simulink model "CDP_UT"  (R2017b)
settings: Solver=FixedStepDiscrete  StartTime=0.0  StopTime=10.0  FixedStep=0.01  RelTol=1e-3  EnableMultiTasking=on
undefined symbols (not defined in the file): ASWTYPE_FALSE, ASWTYPE_TRUE, CaCDP_CellTempNTCVoltTable_mV, CaCDP_CellTempTable_C, CaCDP_CMUPCBTempNTCVoltTable_mV, CaCDP_CMUPCBTempTable_C, CbCDP_DiffBusbarTempStateCheck_flg, CbCDP_DiffCellTempStateCheck_flg, CbCDP_DiffCellVoltStateCheck_flg, CbCDP_IgnorUpdateVld_flg, CbCDP_MaxBusbarTempStateCheck_flg, CbCDP_MaxCellTempStateCheck_flg, CbCDP_MaxCellVoltStateCheck_flg, CbCDP_MinBusbarTempStateCheck_flg, CbCDP_MinCellTempStateCheck_flg, CbCDP_MinCellVoltStateCheck_flg, CcCDP_AFETempConfig_numb, CcCDP_AFETempFltThd_C, CcCDP_AFETempFltThdHys_C, CcCDP_BusbarTempRngFltHiThrd_C, CcCDP_BusbarTempRngFltLowThrd_C, CcCDP_CellDiffFltLevel1_mV, CcCDP_CellDiffFltLevel2_mV, CcCDP_CellDiffFltLevel3_mV, CcCDP_CellTempLowerLimit_C, CcCDP_CellTempRngFltHiThrd_C, CcCDP_CellTempRngFltLowThrd_C, CcCDP_CellTempUpperLimit_C, CcCDP_CellVoltConfig_numb, CcCDP_CellVoltLowerLimit_mV, CcCDP_CellVoltRngHiThrd_mV, CcCDP_CellVoltRngLowThrd_mV, CcCDP_CellVoltUpdateThrd_numb, CcCDP_CellVoltUpperLimit_mV, CcCDP_ChrgMaxCellTempFltLv1Thrd_C, CcCDP_ChrgMaxCellTempFltLv2Thrd_C, CcCDP_ChrgMaxCellTempFltLv3Thrd_C, CcCDP_ChrgMaxCellTempReturnDiff_C, CcCDP_ChrgMinCellTempFltLv1Thrd_C, CcCDP_ChrgMinCellTempFltLv2Thrd_C, CcCDP_ChrgMinCellTempFltLv3Thrd_C, CcCDP_ChrgMinCellTempReturnDiff_C, CcCDP_CMUPCBTempConfig_numb, CcCDP_CMUPCBTempFltThd_C, CcCDP_CMUPCBTempFltThdHys_C, CcCDP_DiffBusbarTempFltLevel1Thrd_C, CcCDP_DiffBusbarTempFltLevel2Thrd_C, CcCDP_DiffBusbarTempReturnDifference_C, CcCDP_DiffCellTempFltLevel1Thrd_C, CcCDP_DiffCellTempFltLevel2Thrd_C, CcCDP_DiffCellTempReturnDifference_C, CcCDP_DiffCellVoltReturnDifference_mV, CcCDP_DiffVoltCheckMaxCellTempCondition_C, CcCDP_DiffVoltCheckMaxCellVoltCondition_mV, CcCDP_DiffVoltCheckMinCellTempCondition_C, CcCDP_DiffVoltCheckMinCellVoltCondition_mV, CcCDP_DiffVoltCheckPackCurrCondition_A, CcCDP_MaxAFETempIniVal_C, CcCDP_MaxBusbarTempFltLevel1Thrd_C, CcCDP_MaxBusbarTempFltLevel2Thrd_C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
libraries: AIWAYS_Powertrain_BMS_lib x148, simulink x8
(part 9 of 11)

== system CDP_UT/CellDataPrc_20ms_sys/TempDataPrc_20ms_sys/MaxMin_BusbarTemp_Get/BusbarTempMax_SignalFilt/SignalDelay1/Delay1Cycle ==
  u : Inport
  Constant2 : Constant  Value=ASWTYPE_FALSE
  Switch : Switch  Criteria=u2 ~= 0  Threshold=1  RndMeth=Zero
  Unit Delay1 : UnitDelay  SampleTime=-1  StateName=StateName
  Unit Delay21 : UnitDelay  InitialCondition=1  SampleTime=-1  StateName=StateName
  y : Outport
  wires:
  Switch/1 -> y/1
  u/1 -> Switch/1, Unit Delay1/1
  Unit Delay1/1 -> Switch/3
  Unit Delay21/1 -> Switch/2
  Constant2/1 -> Unit Delay21/1

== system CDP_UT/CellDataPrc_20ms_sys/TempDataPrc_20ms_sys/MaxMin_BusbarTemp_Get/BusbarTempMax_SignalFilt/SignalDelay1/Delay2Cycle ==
  u : Inport
  Constant2 : Constant  Value=ASWTYPE_FALSE
  Switch : Switch  Criteria=u2 ~= 0  Threshold=1  RndMeth=Zero
  Unit Delay1 : UnitDelay  SampleTime=-1  StateName=StateName
  Unit Delay2 : UnitDelay  InitialCondition=1  SampleTime=-1  StateName=StateName
  Unit Delay21 : UnitDelay  InitialCondition=1  SampleTime=-1  StateName=StateName
  Unit Delay3 : UnitDelay  SampleTime=-1  StateName=StateName
  y : Outport
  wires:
  Unit Delay3/1 -> Switch/3
  Unit Delay2/1 -> Switch/2
  Constant2/1 -> Unit Delay21/1
  Unit Delay21/1 -> Unit Delay2/1
  Unit Delay1/1 -> Unit Delay3/1
  u/1 -> Unit Delay1/1, Switch/1
  Switch/1 -> y/1

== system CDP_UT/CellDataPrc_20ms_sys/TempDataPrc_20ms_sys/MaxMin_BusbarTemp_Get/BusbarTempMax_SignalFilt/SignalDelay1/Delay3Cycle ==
  u : Inport
  Constant2 : Constant  Value=ASWTYPE_FALSE
  Switch : Switch  Criteria=u2 ~= 0  Threshold=1  RndMeth=Zero
  Unit Delay1 : UnitDelay  SampleTime=-1  StateName=StateName
  Unit Delay2 : UnitDelay  InitialCondition=1  SampleTime=-1  StateName=StateName
  Unit Delay21 : UnitDelay  InitialCondition=1  SampleTime=-1  StateName=StateName
  Unit Delay3 : UnitDelay  SampleTime=-1  StateName=StateName
  Unit Delay4 : UnitDelay  InitialCondition=1  SampleTime=-1  StateName=StateName
  Unit Delay5 : UnitDelay  SampleTime=-1  StateName=StateName
  y : Outport
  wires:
  Unit Delay5/1 -> Switch/3
  Unit Delay4/1 -> Switch/2
  Unit Delay3/1 -> Unit Delay5/1
  Unit Delay2/1 -> Unit Delay4/1
  Constant2/1 -> Unit Delay21/1
  Unit Delay21/1 -> Unit Delay2/1
  Unit Delay1/1 -> Unit Delay3/1
  u/1 -> Unit Delay1/1, Switch/1
  Switch/1 -> y/1

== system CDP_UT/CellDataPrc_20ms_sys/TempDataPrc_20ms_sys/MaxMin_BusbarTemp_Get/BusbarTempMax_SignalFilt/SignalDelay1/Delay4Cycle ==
  u : Inport
  Constant2 : Constant  Value=ASWTYPE_FALSE
  Switch : Switch  Criteria=u2 ~= 0  Threshold=1  RndMeth=Zero
  Unit Delay{1,3,5,7} (4 alike) : UnitDelay  SampleTime=-1  StateName=StateName
  Unit Delay{2,4,6,21} (4 alike) : UnitDelay  InitialCondition=1  SampleTime=-1  StateName=StateName
  y : Outport
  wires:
  Unit Delay7/1 -> Switch/3
  Unit Delay6/1 -> Switch/2
  Unit Delay5/1 -> Unit Delay7/1
  Unit Delay4/1 -> Unit Delay6/1
  Unit Delay3/1 -> Unit Delay5/1
  Unit Delay2/1 -> Unit Delay4/1
  Constant2/1 -> Unit Delay21/1
  Unit Delay21/1 -> Unit Delay2/1
  Unit Delay1/1 -> Unit Delay3/1
  u/1 -> Unit Delay1/1, Switch/1
  Switch/1 -> y/1

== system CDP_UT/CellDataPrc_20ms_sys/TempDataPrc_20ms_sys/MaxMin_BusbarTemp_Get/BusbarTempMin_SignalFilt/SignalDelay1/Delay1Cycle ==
  u : Inport
  Constant2 : Constant  Value=ASWTYPE_FALSE
  Switch : Switch  Criteria=u2 ~= 0  Threshold=1  RndMeth=Zero
  Unit Delay1 : UnitDelay  SampleTime=-1  StateName=StateName
  Unit Delay21 : UnitDelay  InitialCondition=1  SampleTime=-1  StateName=StateName
  y : Outport
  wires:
  Constant2/1 -> Unit Delay21/1
  Unit Delay21/1 -> Switch/2
  Unit Delay1/1 -> Switch/3
  u/1 -> Unit Delay1/1, Switch/1
  Switch/1 -> y/1

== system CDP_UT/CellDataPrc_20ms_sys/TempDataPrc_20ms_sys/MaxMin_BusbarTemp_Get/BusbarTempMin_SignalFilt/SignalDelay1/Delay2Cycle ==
  u : Inport
  Constant2 : Constant  Value=ASWTYPE_FALSE
  Switch : Switch  Criteria=u2 ~= 0  Threshold=1  RndMeth=Zero
  Unit Delay1 : UnitDelay  SampleTime=-1  StateName=StateName
  Unit Delay2 : UnitDelay  InitialCondition=1  SampleTime=-1  StateName=StateName
  Unit Delay21 : UnitDelay  InitialCondition=1  SampleTime=-1  StateName=StateName
  Unit Delay3 : UnitDelay  SampleTime=-1  StateName=StateName
  y : Outport
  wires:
  Switch/1 -> y/1
  u/1 -> Switch/1, Unit Delay1/1
  Unit Delay1/1 -> Unit Delay3/1
  Unit Delay21/1 -> Unit Delay2/1
  Constant2/1 -> Unit Delay21/1
  Unit Delay2/1 -> Switch/2
  Unit Delay3/1 -> Switch/3

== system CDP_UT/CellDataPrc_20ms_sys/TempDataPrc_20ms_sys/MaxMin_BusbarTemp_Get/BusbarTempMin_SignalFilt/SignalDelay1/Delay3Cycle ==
  u : Inport
  Constant2 : Constant  Value=ASWTYPE_FALSE
  Switch : Switch  Criteria=u2 ~= 0  Threshold=1  RndMeth=Zero
  Unit Delay1 : UnitDelay  SampleTime=-1  StateName=StateName
  Unit Delay2 : UnitDelay  InitialCondition=1  SampleTime=-1  StateName=StateName
  Unit Delay21 : UnitDelay  InitialCondition=1  SampleTime=-1  StateName=StateName
  Unit Delay3 : UnitDelay  SampleTime=-1  StateName=StateName
  Unit Delay4 : UnitDelay  InitialCondition=1  SampleTime=-1  StateName=StateName
  Unit Delay5 : UnitDelay  SampleTime=-1  StateName=StateName
  y : Outport
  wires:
  Switch/1 -> y/1
  u/1 -> Switch/1, Unit Delay1/1
  Unit Delay1/1 -> Unit Delay3/1
  Unit Delay21/1 -> Unit Delay2/1
  Constant2/1 -> Unit Delay21/1
  Unit Delay2/1 -> Unit Delay4/1
  Unit Delay3/1 -> Unit Delay5/1
  Unit Delay4/1 -> Switch/2
  Unit Delay5/1 -> Switch/3

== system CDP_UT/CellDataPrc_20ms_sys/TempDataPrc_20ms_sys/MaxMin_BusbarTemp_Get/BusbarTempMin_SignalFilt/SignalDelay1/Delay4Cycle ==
  u : Inport
  Constant2 : Constant  Value=ASWTYPE_FALSE
  Switch : Switch  Criteria=u2 ~= 0  Threshold=1  RndMeth=Zero
  Unit Delay{1,3,5,7} (4 alike) : UnitDelay  SampleTime=-1  StateName=StateName
  Unit Delay{2,4,6,21} (4 alike) : UnitDelay  InitialCondition=1  SampleTime=-1  StateName=StateName
  y : Outport
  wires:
  Switch/1 -> y/1
  u/1 -> Switch/1, Unit Delay1/1
  Unit Delay1/1 -> Unit Delay3/1
  Unit Delay21/1 -> Unit Delay2/1
  Constant2/1 -> Unit Delay21/1
  Unit Delay2/1 -> Unit Delay4/1
  Unit Delay3/1 -> Unit Delay5/1
  Unit Delay4/1 -> Unit Delay6/1
  Unit Delay5/1 -> Unit Delay7/1
  Unit Delay6/1 -> Switch/2
  Unit Delay7/1 -> Switch/3

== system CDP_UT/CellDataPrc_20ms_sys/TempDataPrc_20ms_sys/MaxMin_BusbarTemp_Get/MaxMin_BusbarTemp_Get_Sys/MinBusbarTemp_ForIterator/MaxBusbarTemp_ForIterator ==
  LcCDP_IniOutputBusbarTemp_C : Inport
  LcCDP_IniOutputBusbarTempNumb_numb : Inport  Port=2
  LbCDP_IniOutputBusbarTempVld_flg : Inport  Port=3
  Constant3 : Constant  Value=CcCDP_MaxBusbarTempIniVal_C
  Logical Operator : Logic  AllPortsSameDT=off  OutDataTypeStr=boolean
  Relational Operator1 : RelationalOperator  Operator=<=  OutDataTypeStr=boolean
  Switch2 : Switch  Criteria=u2 ~= 0
  Switch3 : Switch  Criteria=u2 ~= 0
  Unit Delay External IC : AIWAYS_Powertrain_BMS_lib/Delay Blocks/Unit Delay External IC
  Unit Delay External IC2 : AIWAYS_Powertrain_BMS_lib/Delay Blocks/Unit Delay External IC
  Unit Delay3 : UnitDelay  SampleTime=-1  StateName=StateName
  LcCDP_MaxBusbarTempNumb_numb : Outport
  LcCDP_MaxBusbarTemp_C : Outport  Port=2
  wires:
  LbCDP_IniOutputBusbarTempVld_flg/1 -> Logical Operator/1
  [LbCDP_BusbarTempMaxSelction_flg] -> Logical Operator/2
  Switch2/1 -> Unit Delay External IC2/1, LcCDP_MaxBusbarTemp_C/1, Unit Delay External IC/1  "LcCDP_MaxBusbarTemp_C"
  Unit Delay External IC/1 -> Relational Operator1/1
  Relational Operator1/1 -> [LbCDP_BusbarTempMaxSelction_flg]  "LbCDP_BusbarTempMaxSelction_flg"
  LcCDP_IniOutputBusbarTempNumb_numb/1 -> Switch3/1
  LcCDP_IniOutputBusbarTemp_C/1 -> Switch2/1, Relational Operator1/2, Unit Delay External IC/2
  Unit Delay External IC2/1 -> Switch2/3
  Logical Operator/1 -> Switch2/2, Switch3/2
  Unit Delay3/1 -> Switch3/3
  Switch3/1 -> Unit Delay3/1, LcCDP_MaxBusbarTempNumb_numb/1  "LcCDP_MaxBusbarTempNumb_numb"
  Constant3/1 -> Unit Delay External IC2/2

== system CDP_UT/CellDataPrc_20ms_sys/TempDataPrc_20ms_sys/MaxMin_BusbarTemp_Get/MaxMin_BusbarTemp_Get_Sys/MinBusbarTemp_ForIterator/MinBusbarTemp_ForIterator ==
  LcCDP_IniOutputBusbarTemp_C : Inport
  LcCDP_IniOutputBusbarTempNumb_numb : Inport  Port=2
  LbCDP_IniOutputBusbarTempVld_flg : Inport  Port=3
  Constant3 : Constant  Value=CcCDP_MinBusbarTempIniVal_C
  Logical Operator : Logic  AllPortsSameDT=off  OutDataTypeStr=boolean
  Relational Operator3 : RelationalOperator  OutDataTypeStr=boolean
  Switch : Switch  Criteria=u2 ~= 0
  Switch1 : Switch  Criteria=u2 ~= 0
  Unit Delay External IC1 : AIWAYS_Powertrain_BMS_lib/Delay Blocks/Unit Delay External IC
  Unit Delay External IC2 : AIWAYS_Powertrain_BMS_lib/Delay Blocks/Unit Delay External IC
  Unit Delay1 : UnitDelay  SampleTime=-1  StateName=StateName
  LcCDP_MinBusbarTemp_C : Outport
  LcCDP_MinBusbarTempNumb_numb : Outport  Port=2
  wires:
  [LbCDP_BusbarTempMinSelction_flg] -> Logical Operator/2
  LbCDP_IniOutputBusbarTempVld_flg/1 -> Logical Operator/1
  Unit Delay External IC1/1 -> Relational Operator3/1
  Switch/1 -> Unit Delay External IC2/1, LcCDP_MinBusbarTemp_C/1, Unit Delay External IC1/1  "LcCDP_MinBusbarTemp_C"
  LcCDP_IniOutputBusbarTemp_C/1 -> Switch/1, Relational Operator3/2, Unit Delay External IC1/2
  Logical Operator/1 -> Switch1/2, Switch/2
  Unit Delay External IC2/1 -> Switch/3
  Relational Operator3/1 -> [LbCDP_BusbarTempMinSelction_flg]  "LbCDP_BusbarTempMinSelction_flg"
  Unit Delay1/1 -> Switch1/3
  LcCDP_IniOutputBusbarTempNumb_numb/1 -> Switch1/1
  Switch1/1 -> Unit Delay1/1, LcCDP_MinBusbarTempNumb_numb/1  "LcCDP_MinBusbarTempNumb_numb"
  Constant3/1 -> Unit Delay External IC2/2

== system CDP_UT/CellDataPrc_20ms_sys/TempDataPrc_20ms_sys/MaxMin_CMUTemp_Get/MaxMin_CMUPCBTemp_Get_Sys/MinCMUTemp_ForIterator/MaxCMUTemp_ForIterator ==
  LcCDP_IniOutputCMUPCBTemp_C : Inport
  LcCDP_IniOutputCMUPCBTempNumb_numb : Inport  Port=2
  LbCDP_IniOutputCMUPCBTempVld_flg : Inport  Port=3
  Constant3 : Constant  Value=CcCDP_MaxCMUPCBTempIniVal_C
  Logical Operator : Logic  AllPortsSameDT=off  OutDataTypeStr=boolean
  Relational Operator1 : RelationalOperator  Operator=<=  OutDataTypeStr=boolean
  Switch2 : Switch  Criteria=u2 ~= 0
  Switch3 : Switch  Criteria=u2 ~= 0
  Unit Delay External IC : AIWAYS_Powertrain_BMS_lib/Delay Blocks/Unit Delay External IC
  Unit Delay External IC2 : AIWAYS_Powertrain_BMS_lib/Delay Blocks/Unit Delay External IC
  Unit Delay3 : UnitDelay  SampleTime=-1  StateName=StateName
  LcCDP_MaxCMUPCBTempNumb_numb : Outport
  LcCDP_MaxCMUPCBTemp_C : Outport  Port=2
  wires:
  Switch3/1 -> LcCDP_MaxCMUPCBTempNumb_numb/1, Unit Delay3/1  "LcCDP_MaxCMUPCBTempNumb_numb"
  Unit Delay3/1 -> Switch3/3
  Logical Operator/1 -> Switch3/2, Switch2/2
  Unit Delay External IC2/1 -> Switch2/3
  LcCDP_IniOutputCMUPCBTemp_C/1 -> Unit Delay External IC/2, Relational Operator1/2, Switch2/1
  LcCDP_IniOutputCMUPCBTempNumb_numb/1 -> Switch3/1
  Relational Operator1/1 -> [LbCDP_CMUPCBTempMaxSelction_flg]  "LbCDP_CMUPCBTempMaxSelction_flg"
  Unit Delay External IC/1 -> Relational Operator1/1
  Switch2/1 -> Unit Delay External IC2/1, Unit Delay External IC/1, LcCDP_MaxCMUPCBTemp_C/1  "LcCDP_MaxCMUPCBTemp_C"
  [LbCDP_CMUPCBTempMaxSelction_flg] -> Logical Operator/2
  LbCDP_IniOutputCMUPCBTempVld_flg/1 -> Logical Operator/1
  Constant3/1 -> Unit Delay External IC2/2

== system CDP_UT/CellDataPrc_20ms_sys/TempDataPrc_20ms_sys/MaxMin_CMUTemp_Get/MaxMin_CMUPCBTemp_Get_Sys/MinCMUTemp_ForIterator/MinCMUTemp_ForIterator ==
  LcCDP_IniOutputCMUPCBTemp_C : Inport
  LcCDP_IniOutputCMUPCBTempNumb_numb : Inport  Port=2
  LbCDP_IniOutputCMUPCBTempVld_flg : Inport  Port=3
  Constant3 : Constant  Value=CcCDP_MinCMUPCBTempIniVal_C
  Logical Operator : Logic  AllPortsSameDT=off  OutDataTypeStr=boolean
  Relational Operator3 : RelationalOperator  OutDataTypeStr=boolean
  Switch : Switch  Criteria=u2 ~= 0
  Switch1 : Switch  Criteria=u2 ~= 0
  Unit Delay External IC1 : AIWAYS_Powertrain_BMS_lib/Delay Blocks/Unit Delay External IC
  Unit Delay External IC2 : AIWAYS_Powertrain_BMS_lib/Delay Blocks/Unit Delay External IC
  Unit Delay1 : UnitDelay  SampleTime=-1  StateName=StateName
  LcCDP_MinCMUPCBTemp_C : Outport
  LcCDP_MinCMUPCBTempNumb_numb : Outport  Port=2
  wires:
  Switch1/1 -> LcCDP_MinCMUPCBTempNumb_numb/1, Unit Delay1/1  "LcCDP_MinCMUPCBTempNumb_numb"
  LcCDP_IniOutputCMUPCBTempNumb_numb/1 -> Switch1/1
  Unit Delay1/1 -> Switch1/3
  Relational Operator3/1 -> [LbCDP_CMUPCBTempMinSelction_flg]  "LbCDP_CMUPCBTempMinSelction_flg"
  Unit Delay External IC2/1 -> Switch/3
  Logical Operator/1 -> Switch/2, Switch1/2
  LcCDP_IniOutputCMUPCBTemp_C/1 -> Unit Delay External IC1/2, Relational Operator3/2, Switch/1
  Switch/1 -> Unit Delay External IC1/1, Unit Delay External IC2/1, LcCDP_MinCMUPCBTemp_C/1  "LcCDP_MinCMUPCBTemp_C"
  Unit Delay External IC1/1 -> Relational Operator3/1
  LbCDP_IniOutputCMUPCBTempVld_flg/1 -> Logical Operator/1
  [LbCDP_CMUPCBTempMinSelction_flg] -> Logical Operator/2
  Constant3/1 -> Unit Delay External IC2/2

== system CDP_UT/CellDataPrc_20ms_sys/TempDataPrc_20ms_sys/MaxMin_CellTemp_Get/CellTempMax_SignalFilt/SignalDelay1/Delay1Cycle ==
  u : Inport
  Constant2 : Constant  Value=ASWTYPE_FALSE
  Switch : Switch  Criteria=u2 ~= 0  Threshold=1  RndMeth=Zero
  Unit Delay1 : UnitDelay  SampleTime=-1  StateName=StateName
  Unit Delay21 : UnitDelay  InitialCondition=1  SampleTime=-1  StateName=StateName
  y : Outport
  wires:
  Switch/1 -> y/1
  u/1 -> Switch/1, Unit Delay1/1
  Unit Delay1/1 -> Switch/3
  Unit Delay21/1 -> Switch/2
  Constant2/1 -> Unit Delay21/1

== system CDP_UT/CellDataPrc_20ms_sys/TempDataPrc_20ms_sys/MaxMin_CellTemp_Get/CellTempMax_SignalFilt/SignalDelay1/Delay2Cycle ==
  u : Inport
  Constant2 : Constant  Value=ASWTYPE_FALSE
  Switch : Switch  Criteria=u2 ~= 0  Threshold=1  RndMeth=Zero
  Unit Delay1 : UnitDelay  SampleTime=-1  StateName=StateName
  Unit Delay2 : UnitDelay  InitialCondition=1  SampleTime=-1  StateName=StateName
  Unit Delay21 : UnitDelay  InitialCondition=1  SampleTime=-1  StateName=StateName
  Unit Delay3 : UnitDelay  SampleTime=-1  StateName=StateName
  y : Outport
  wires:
  Unit Delay3/1 -> Switch/3
  Unit Delay2/1 -> Switch/2
  Constant2/1 -> Unit Delay21/1
  Unit Delay21/1 -> Unit Delay2/1
  Unit Delay1/1 -> Unit Delay3/1
  u/1 -> Unit Delay1/1, Switch/1
  Switch/1 -> y/1

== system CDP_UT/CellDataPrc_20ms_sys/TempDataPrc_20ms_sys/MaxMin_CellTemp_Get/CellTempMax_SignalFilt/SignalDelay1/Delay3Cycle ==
  u : Inport
  Constant2 : Constant  Value=ASWTYPE_FALSE
  Switch : Switch  Criteria=u2 ~= 0  Threshold=1  RndMeth=Zero
  Unit Delay1 : UnitDelay  SampleTime=-1  StateName=StateName
  Unit Delay2 : UnitDelay  InitialCondition=1  SampleTime=-1  StateName=StateName
  Unit Delay21 : UnitDelay  InitialCondition=1  SampleTime=-1  StateName=StateName
  Unit Delay3 : UnitDelay  SampleTime=-1  StateName=StateName
  Unit Delay4 : UnitDelay  InitialCondition=1  SampleTime=-1  StateName=StateName
  Unit Delay5 : UnitDelay  SampleTime=-1  StateName=StateName
  y : Outport
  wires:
  Unit Delay5/1 -> Switch/3
  Unit Delay4/1 -> Switch/2
  Unit Delay3/1 -> Unit Delay5/1
  Unit Delay2/1 -> Unit Delay4/1
  Constant2/1 -> Unit Delay21/1
  Unit Delay21/1 -> Unit Delay2/1
  Unit Delay1/1 -> Unit Delay3/1
  u/1 -> Unit Delay1/1, Switch/1
  Switch/1 -> y/1

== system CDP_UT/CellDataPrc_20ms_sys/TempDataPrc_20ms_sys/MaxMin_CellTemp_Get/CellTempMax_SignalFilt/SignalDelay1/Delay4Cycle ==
  u : Inport
  Constant2 : Constant  Value=ASWTYPE_FALSE
  Switch : Switch  Criteria=u2 ~= 0  Threshold=1  RndMeth=Zero
  Unit Delay{1,3,5,7} (4 alike) : UnitDelay  SampleTime=-1  StateName=StateName
  Unit Delay{2,4,6,21} (4 alike) : UnitDelay  InitialCondition=1  SampleTime=-1  StateName=StateName
  y : Outport
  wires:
  Unit Delay7/1 -> Switch/3
  Unit Delay6/1 -> Switch/2
  Unit Delay5/1 -> Unit Delay7/1
  Unit Delay4/1 -> Unit Delay6/1
  Unit Delay3/1 -> Unit Delay5/1
  Unit Delay2/1 -> Unit Delay4/1
  Constant2/1 -> Unit Delay21/1
  Unit Delay21/1 -> Unit Delay2/1
  Unit Delay1/1 -> Unit Delay3/1
  u/1 -> Unit Delay1/1, Switch/1
  Switch/1 -> y/1

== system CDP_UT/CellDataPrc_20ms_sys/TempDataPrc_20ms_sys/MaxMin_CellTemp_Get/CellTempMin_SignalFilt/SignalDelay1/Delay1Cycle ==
  u : Inport
  Constant2 : Constant  Value=ASWTYPE_FALSE
  Switch : Switch  Criteria=u2 ~= 0  Threshold=1  RndMeth=Zero
  Unit Delay1 : UnitDelay  SampleTime=-1  StateName=StateName
  Unit Delay21 : UnitDelay  InitialCondition=1  SampleTime=-1  StateName=StateName
  y : Outport
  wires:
  Constant2/1 -> Unit Delay21/1
  Unit Delay21/1 -> Switch/2
  Unit Delay1/1 -> Switch/3
  u/1 -> Unit Delay1/1, Switch/1
  Switch/1 -> y/1

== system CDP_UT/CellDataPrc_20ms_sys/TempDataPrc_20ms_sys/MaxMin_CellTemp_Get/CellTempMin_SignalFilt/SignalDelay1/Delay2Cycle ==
  u : Inport
  Constant2 : Constant  Value=ASWTYPE_FALSE
  Switch : Switch  Criteria=u2 ~= 0  Threshold=1  RndMeth=Zero
  Unit Delay1 : UnitDelay  SampleTime=-1  StateName=StateName
  Unit Delay2 : UnitDelay  InitialCondition=1  SampleTime=-1  StateName=StateName
  Unit Delay21 : UnitDelay  InitialCondition=1  SampleTime=-1  StateName=StateName
  Unit Delay3 : UnitDelay  SampleTime=-1  StateName=StateName
  y : Outport
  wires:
  Switch/1 -> y/1
  u/1 -> Switch/1, Unit Delay1/1
  Unit Delay1/1 -> Unit Delay3/1
  Unit Delay21/1 -> Unit Delay2/1
  Constant2/1 -> Unit Delay21/1
  Unit Delay2/1 -> Switch/2
  Unit Delay3/1 -> Switch/3

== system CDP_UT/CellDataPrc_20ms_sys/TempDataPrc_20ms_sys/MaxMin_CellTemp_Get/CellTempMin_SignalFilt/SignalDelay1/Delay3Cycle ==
  u : Inport
  Constant2 : Constant  Value=ASWTYPE_FALSE
  Switch : Switch  Criteria=u2 ~= 0  Threshold=1  RndMeth=Zero
  Unit Delay1 : UnitDelay  SampleTime=-1  StateName=StateName
  Unit Delay2 : UnitDelay  InitialCondition=1  SampleTime=-1  StateName=StateName
  Unit Delay21 : UnitDelay  InitialCondition=1  SampleTime=-1  StateName=StateName
  Unit Delay3 : UnitDelay  SampleTime=-1  StateName=StateName
  Unit Delay4 : UnitDelay  InitialCondition=1  SampleTime=-1  StateName=StateName
  Unit Delay5 : UnitDelay  SampleTime=-1  StateName=StateName
  y : Outport
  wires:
  Switch/1 -> y/1
  u/1 -> Switch/1, Unit Delay1/1
  Unit Delay1/1 -> Unit Delay3/1
  Unit Delay21/1 -> Unit Delay2/1
  Constant2/1 -> Unit Delay21/1
  Unit Delay2/1 -> Unit Delay4/1
  Unit Delay3/1 -> Unit Delay5/1
  Unit Delay4/1 -> Switch/2
  Unit Delay5/1 -> Switch/3

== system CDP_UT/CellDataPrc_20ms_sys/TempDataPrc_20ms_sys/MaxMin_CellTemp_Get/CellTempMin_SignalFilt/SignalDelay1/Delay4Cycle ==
  u : Inport
  Constant2 : Constant  Value=ASWTYPE_FALSE
  Switch : Switch  Criteria=u2 ~= 0  Threshold=1  RndMeth=Zero
  Unit Delay{1,3,5,7} (4 alike) : UnitDelay  SampleTime=-1  StateName=StateName
  Unit Delay{2,4,6,21} (4 alike) : UnitDelay  InitialCondition=1  SampleTime=-1  StateName=StateName
  y : Outport
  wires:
  Switch/1 -> y/1
  u/1 -> Switch/1, Unit Delay1/1
  Unit Delay1/1 -> Unit Delay3/1
  Unit Delay21/1 -> Unit Delay2/1
  Constant2/1 -> Unit Delay21/1
  Unit Delay2/1 -> Unit Delay4/1
  Unit Delay3/1 -> Unit Delay5/1
  Unit Delay4/1 -> Unit Delay6/1
  Unit Delay5/1 -> Unit Delay7/1
  Unit Delay6/1 -> Switch/2
  Unit Delay7/1 -> Switch/3

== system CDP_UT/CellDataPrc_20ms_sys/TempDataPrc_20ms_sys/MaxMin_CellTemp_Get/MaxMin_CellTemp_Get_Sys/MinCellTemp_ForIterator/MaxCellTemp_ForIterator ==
  LcCDP_IniOutputCellTemp_C : Inport
  LcCDP_IniOutputCellTempNumb_numb : Inport  Port=2
  LbCDP_IniOutputCellTempVld_flg : Inport  Port=3
  Constant3 : Constant  Value=CcCDP_MaxCellTempIniVal_C
  Logical Operator : Logic  AllPortsSameDT=off  OutDataTypeStr=boolean
  Relational Operator1 : RelationalOperator  Operator=<=  OutDataTypeStr=boolean
  Switch2 : Switch  Criteria=u2 ~= 0
  Switch3 : Switch  Criteria=u2 ~= 0
  Unit Delay External IC : AIWAYS_Powertrain_BMS_lib/Delay Blocks/Unit Delay External IC
  Unit Delay External IC2 : AIWAYS_Powertrain_BMS_lib/Delay Blocks/Unit Delay External IC
  Unit Delay3 : UnitDelay  SampleTime=-1  StateName=StateName
  LcCDP_MaxCellTempNumb_numb : Outport
  LcCDP_MaxCellTemp_C : Outport  Port=2
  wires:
  Switch3/1 -> LcCDP_MaxCellTempNumb_numb/1, Unit Delay3/1  "LcCDP_MaxCellTempNumb_numb"
  Unit Delay3/1 -> Switch3/3
  Logical Operator/1 -> Switch3/2, Switch2/2
  Unit Delay External IC2/1 -> Switch2/3
  LcCDP_IniOutputCellTemp_C/1 -> Unit Delay External IC/2, Relational Operator1/2, Switch2/1
  LcCDP_IniOutputCellTempNumb_numb/1 -> Switch3/1
  Relational Operator1/1 -> [LbCDP_CellTempMaxSelction_flg]  "LbCDP_CellTempMaxSelction_flg"
  Unit Delay External IC/1 -> Relational Operator1/1
  Switch2/1 -> Unit Delay External IC2/1, Unit Delay External IC/1, LcCDP_MaxCellTemp_C/1  "LcCDP_MaxCellTemp_C"
  [LbCDP_CellTempMaxSelction_flg] -> Logical Operator/2
  LbCDP_IniOutputCellTempVld_flg/1 -> Logical Operator/1
  Constant3/1 -> Unit Delay External IC2/2

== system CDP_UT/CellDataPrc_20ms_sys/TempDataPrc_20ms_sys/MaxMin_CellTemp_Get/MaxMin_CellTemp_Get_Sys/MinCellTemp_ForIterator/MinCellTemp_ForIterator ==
  LcCDP_IniOutputCellTemp_C : Inport
  LcCDP_IniOutputCellTempNumb_numb : Inport  Port=2
  LbCDP_IniOutputCellTempVld_flg : Inport  Port=3
  Constant3 : Constant  Value=CcCDP_MinCellTempIniVal_C
  Logical Operator : Logic  AllPortsSameDT=off  OutDataTypeStr=boolean
  Relational Operator3 : RelationalOperator  OutDataTypeStr=boolean
  Switch : Switch  Criteria=u2 ~= 0
  Switch1 : Switch  Criteria=u2 ~= 0
  Unit Delay External IC1 : AIWAYS_Powertrain_BMS_lib/Delay Blocks/Unit Delay External IC
  Unit Delay External IC2 : AIWAYS_Powertrain_BMS_lib/Delay Blocks/Unit Delay External IC
  Unit Delay1 : UnitDelay  SampleTime=-1  StateName=StateName
  LcCDP_MinCellTemp_C : Outport
  LcCDP_MinCellTempNumb_numb : Outport  Port=2
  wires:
  Switch1/1 -> LcCDP_MinCellTempNumb_numb/1, Unit Delay1/1  "LcCDP_MinCellTempNumb_numb"
  LcCDP_IniOutputCellTempNumb_numb/1 -> Switch1/1
  Unit Delay1/1 -> Switch1/3
  Relational Operator3/1 -> [LbCDP_CellTempMinSelction_flg]  "LbCDP_CellTempMinSelction_flg"
  Unit Delay External IC2/1 -> Switch/3
  Logical Operator/1 -> Switch/2, Switch1/2
  LcCDP_IniOutputCellTemp_C/1 -> Unit Delay External IC1/2, Relational Operator3/2, Switch/1
  Switch/1 -> Unit Delay External IC1/1, Unit Delay External IC2/1, LcCDP_MinCellTemp_C/1  "LcCDP_MinCellTemp_C"
  Unit Delay External IC1/1 -> Relational Operator3/1
  LbCDP_IniOutputCellTempVld_flg/1 -> Logical Operator/1
  [LbCDP_CellTempMinSelction_flg] -> Logical Operator/2
  Constant3/1 -> Unit Delay External IC2/2

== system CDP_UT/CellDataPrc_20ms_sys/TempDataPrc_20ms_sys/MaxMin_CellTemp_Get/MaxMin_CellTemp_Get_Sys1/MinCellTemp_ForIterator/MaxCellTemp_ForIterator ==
  LcCDP_IniOutputCellTemp_C : Inport
  LcCDP_IniOutputCellTempNumb_numb : Inport  Port=2
  LbCDP_IniOutputCellTempVld_flg : Inport  Port=3
  Constant3 : Constant  Value=CcCDP_MaxCellTempIniVal_C
  Logical Operator : Logic  AllPortsSameDT=off  OutDataTypeStr=boolean
  Relational Operator1 : RelationalOperator  Operator=<=  OutDataTypeStr=boolean
  Switch2 : Switch  Criteria=u2 ~= 0
  Switch3 : Switch  Criteria=u2 ~= 0
  Unit Delay External IC : AIWAYS_Powertrain_BMS_lib/Delay Blocks/Unit Delay External IC
  Unit Delay External IC2 : AIWAYS_Powertrain_BMS_lib/Delay Blocks/Unit Delay External IC
  Unit Delay3 : UnitDelay  SampleTime=-1  StateName=StateName
  LcCDP_MaxCellTempNumb_numb : Outport
  LcCDP_MaxCellTemp_C : Outport  Port=2
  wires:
  Switch3/1 -> LcCDP_MaxCellTempNumb_numb/1, Unit Delay3/1  "LcCDP_MaxCellTempNumb_numb"
  Unit Delay3/1 -> Switch3/3
  Logical Operator/1 -> Switch3/2, Switch2/2
  Unit Delay External IC2/1 -> Switch2/3
  LcCDP_IniOutputCellTemp_C/1 -> Unit Delay External IC/2, Relational Operator1/2, Switch2/1
  LcCDP_IniOutputCellTempNumb_numb/1 -> Switch3/1
  Relational Operator1/1 -> [LbCDP_CellTempMaxSelction_flg]  "LbCDP_CellTempMaxSelction_flg"
  Unit Delay External IC/1 -> Relational Operator1/1
  Switch2/1 -> Unit Delay External IC2/1, Unit Delay External IC/1, LcCDP_MaxCellTemp_C/1  "LcCDP_MaxCellTemp_C"
  [LbCDP_CellTempMaxSelction_flg] -> Logical Operator/2
  LbCDP_IniOutputCellTempVld_flg/1 -> Logical Operator/1
  Constant3/1 -> Unit Delay External IC2/2

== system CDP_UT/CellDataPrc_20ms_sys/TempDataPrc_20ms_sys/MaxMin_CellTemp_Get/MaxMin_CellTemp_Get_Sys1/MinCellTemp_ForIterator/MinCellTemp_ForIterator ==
  LcCDP_IniOutputCellTemp_C : Inport
  LcCDP_IniOutputCellTempNumb_numb : Inport  Port=2
  LbCDP_IniOutputCellTempVld_flg : Inport  Port=3
  Constant3 : Constant  Value=CcCDP_MinCellTempIniVal_C
  Logical Operator : Logic  AllPortsSameDT=off  OutDataTypeStr=boolean
  Relational Operator3 : RelationalOperator  OutDataTypeStr=boolean
  Switch : Switch  Criteria=u2 ~= 0
  Switch1 : Switch  Criteria=u2 ~= 0
  Unit Delay External IC1 : AIWAYS_Powertrain_BMS_lib/Delay Blocks/Unit Delay External IC
  Unit Delay External IC2 : AIWAYS_Powertrain_BMS_lib/Delay Blocks/Unit Delay External IC
  Unit Delay1 : UnitDelay  SampleTime=-1  StateName=StateName
  LcCDP_MinCellTemp_C : Outport
  LcCDP_MinCellTempNumb_numb : Outport  Port=2
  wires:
  Switch1/1 -> LcCDP_MinCellTempNumb_numb/1, Unit Delay1/1  "LcCDP_MinCellTempNumb_numb"
  LcCDP_IniOutputCellTempNumb_numb/1 -> Switch1/1
  Unit Delay1/1 -> Switch1/3
  Relational Operator3/1 -> [LbCDP_CellTempMinSelction_flg]  "LbCDP_CellTempMinSelction_flg"
  Unit Delay External IC2/1 -> Switch/3
  Logical Operator/1 -> Switch/2, Switch1/2
  LcCDP_IniOutputCellTemp_C/1 -> Unit Delay External IC1/2, Relational Operator3/2, Switch/1
  Switch/1 -> Unit Delay External IC1/1, Unit Delay External IC2/1, LcCDP_MinCellTemp_C/1  "LcCDP_MinCellTemp_C"
  Unit Delay External IC1/1 -> Relational Operator3/1
  LbCDP_IniOutputCellTempVld_flg/1 -> Logical Operator/1
  [LbCDP_CellTempMinSelction_flg] -> Logical Operator/2
  Constant3/1 -> Unit Delay External IC2/2

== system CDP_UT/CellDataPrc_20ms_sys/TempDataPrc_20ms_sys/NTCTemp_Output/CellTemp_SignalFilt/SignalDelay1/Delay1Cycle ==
  u : Inport
  Constant2 : Constant  Value=ASWTYPE_FALSE
  Switch : Switch  Criteria=u2 ~= 0  Threshold=1  RndMeth=Zero
  Unit Delay1 : UnitDelay  SampleTime=-1  StateName=StateName
  Unit Delay21 : UnitDelay  InitialCondition=1  SampleTime=-1  StateName=StateName
  y : Outport
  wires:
  Switch/1 -> y/1
  u/1 -> Switch/1, Unit Delay1/1
  Unit Delay1/1 -> Switch/3
  Unit Delay21/1 -> Switch/2
  Constant2/1 -> Unit Delay21/1

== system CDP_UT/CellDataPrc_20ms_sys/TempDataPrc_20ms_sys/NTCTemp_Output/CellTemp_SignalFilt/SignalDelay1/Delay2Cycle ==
  u : Inport
  Constant2 : Constant  Value=ASWTYPE_FALSE
  Switch : Switch  Criteria=u2 ~= 0  Threshold=1  RndMeth=Zero
  Unit Delay1 : UnitDelay  SampleTime=-1  StateName=StateName
  Unit Delay2 : UnitDelay  InitialCondition=1  SampleTime=-1  StateName=StateName
  Unit Delay21 : UnitDelay  InitialCondition=1  SampleTime=-1  StateName=StateName
  Unit Delay3 : UnitDelay  SampleTime=-1  StateName=StateName
  y : Outport
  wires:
  Unit Delay3/1 -> Switch/3
  Unit Delay2/1 -> Switch/2
  Constant2/1 -> Unit Delay21/1
  Unit Delay21/1 -> Unit Delay2/1
  Unit Delay1/1 -> Unit Delay3/1
  u/1 -> Unit Delay1/1, Switch/1
  Switch/1 -> y/1

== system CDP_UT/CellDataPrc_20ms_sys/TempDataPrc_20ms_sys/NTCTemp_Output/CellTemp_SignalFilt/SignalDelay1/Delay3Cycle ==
  u : Inport
  Constant2 : Constant  Value=ASWTYPE_FALSE
  Switch : Switch  Criteria=u2 ~= 0  Threshold=1  RndMeth=Zero
  Unit Delay1 : UnitDelay  SampleTime=-1  StateName=StateName
  Unit Delay2 : UnitDelay  InitialCondition=1  SampleTime=-1  StateName=StateName
  Unit Delay21 : UnitDelay  InitialCondition=1  SampleTime=-1  StateName=StateName
  Unit Delay3 : UnitDelay  SampleTime=-1  StateName=StateName
  Unit Delay4 : UnitDelay  InitialCondition=1  SampleTime=-1  StateName=StateName
  Unit Delay5 : UnitDelay  SampleTime=-1  StateName=StateName
  y : Outport
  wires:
  Unit Delay5/1 -> Switch/3
  Unit Delay4/1 -> Switch/2
  Unit Delay3/1 -> Unit Delay5/1
  Unit Delay2/1 -> Unit Delay4/1
  Constant2/1 -> Unit Delay21/1
  Unit Delay21/1 -> Unit Delay2/1
  Unit Delay1/1 -> Unit Delay3/1
  u/1 -> Unit Delay1/1, Switch/1
  Switch/1 -> y/1

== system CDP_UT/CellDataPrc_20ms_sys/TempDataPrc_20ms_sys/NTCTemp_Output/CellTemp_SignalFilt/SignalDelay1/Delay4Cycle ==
  u : Inport
  Constant2 : Constant  Value=ASWTYPE_FALSE
  Switch : Switch  Criteria=u2 ~= 0  Threshold=1  RndMeth=Zero
  Unit Delay{1,3,5,7} (4 alike) : UnitDelay  SampleTime=-1  StateName=StateName
  Unit Delay{2,4,6,21} (4 alike) : UnitDelay  InitialCondition=1  SampleTime=-1  StateName=StateName
  y : Outport
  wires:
  Unit Delay7/1 -> Switch/3
  Unit Delay6/1 -> Switch/2
  Unit Delay5/1 -> Unit Delay7/1
  Unit Delay4/1 -> Unit Delay6/1
  Unit Delay3/1 -> Unit Delay5/1
  Unit Delay2/1 -> Unit Delay4/1
  Constant2/1 -> Unit Delay21/1
  Unit Delay21/1 -> Unit Delay2/1
  Unit Delay1/1 -> Unit Delay3/1
  u/1 -> Unit Delay1/1, Switch/1
  Switch/1 -> y/1

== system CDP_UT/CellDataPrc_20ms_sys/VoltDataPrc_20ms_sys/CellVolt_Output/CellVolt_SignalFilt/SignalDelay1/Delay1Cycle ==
  u : Inport
  Constant2 : Constant  Value=ASWTYPE_FALSE
  Switch : Switch  Criteria=u2 ~= 0  Threshold=1  RndMeth=Zero
  Unit Delay1 : UnitDelay  SampleTime=-1  StateName=StateName
  Unit Delay21 : UnitDelay  InitialCondition=1  SampleTime=-1  StateName=StateName
  y : Outport
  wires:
  Switch/1 -> y/1
  u/1 -> Switch/1, Unit Delay1/1
  Unit Delay1/1 -> Switch/3
  Unit Delay21/1 -> Switch/2
  Constant2/1 -> Unit Delay21/1

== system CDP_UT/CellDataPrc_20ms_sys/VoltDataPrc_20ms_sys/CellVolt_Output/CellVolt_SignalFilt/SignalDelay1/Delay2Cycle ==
  u : Inport
  Constant2 : Constant  Value=ASWTYPE_FALSE
  Switch : Switch  Criteria=u2 ~= 0  Threshold=1  RndMeth=Zero
  Unit Delay1 : UnitDelay  SampleTime=-1  StateName=StateName
  Unit Delay2 : UnitDelay  InitialCondition=1  SampleTime=-1  StateName=StateName
  Unit Delay21 : UnitDelay  InitialCondition=1  SampleTime=-1  StateName=StateName
  Unit Delay3 : UnitDelay  SampleTime=-1  StateName=StateName
  y : Outport
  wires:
  Unit Delay3/1 -> Switch/3
  Unit Delay2/1 -> Switch/2
  Constant2/1 -> Unit Delay21/1
  Unit Delay21/1 -> Unit Delay2/1
  Unit Delay1/1 -> Unit Delay3/1
  u/1 -> Unit Delay1/1, Switch/1
  Switch/1 -> y/1

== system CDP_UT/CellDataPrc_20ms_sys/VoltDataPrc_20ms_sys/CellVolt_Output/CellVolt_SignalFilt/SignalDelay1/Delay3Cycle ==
  u : Inport
  Constant2 : Constant  Value=ASWTYPE_FALSE
  Switch : Switch  Criteria=u2 ~= 0  Threshold=1  RndMeth=Zero
  Unit Delay1 : UnitDelay  SampleTime=-1  StateName=StateName
  Unit Delay2 : UnitDelay  InitialCondition=1  SampleTime=-1  StateName=StateName
  Unit Delay21 : UnitDelay  InitialCondition=1  SampleTime=-1  StateName=StateName
  Unit Delay3 : UnitDelay  SampleTime=-1  StateName=StateName
  Unit Delay4 : UnitDelay  InitialCondition=1  SampleTime=-1  StateName=StateName
  Unit Delay5 : UnitDelay  SampleTime=-1  StateName=StateName
  y : Outport
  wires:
  Unit Delay5/1 -> Switch/3
  Unit Delay4/1 -> Switch/2
  Unit Delay3/1 -> Unit Delay5/1
  Unit Delay2/1 -> Unit Delay4/1
  Constant2/1 -> Unit Delay21/1
  Unit Delay21/1 -> Unit Delay2/1
  Unit Delay1/1 -> Unit Delay3/1
  u/1 -> Unit Delay1/1, Switch/1
  Switch/1 -> y/1

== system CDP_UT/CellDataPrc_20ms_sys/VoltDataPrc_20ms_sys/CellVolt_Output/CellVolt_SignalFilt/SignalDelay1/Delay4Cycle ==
  u : Inport
  Constant2 : Constant  Value=ASWTYPE_FALSE
  Switch : Switch  Criteria=u2 ~= 0  Threshold=1  RndMeth=Zero
  Unit Delay{1,3,5,7} (4 alike) : UnitDelay  SampleTime=-1  StateName=StateName
  Unit Delay{2,4,6,21} (4 alike) : UnitDelay  InitialCondition=1  SampleTime=-1  StateName=StateName
  y : Outport
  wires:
  Unit Delay7/1 -> Switch/3
  Unit Delay6/1 -> Switch/2
  Unit Delay5/1 -> Unit Delay7/1
  Unit Delay4/1 -> Unit Delay6/1
  Unit Delay3/1 -> Unit Delay5/1
  Unit Delay2/1 -> Unit Delay4/1
  Constant2/1 -> Unit Delay21/1
  Unit Delay21/1 -> Unit Delay2/1
  Unit Delay1/1 -> Unit Delay3/1
  u/1 -> Unit Delay1/1, Switch/1
  Switch/1 -> y/1

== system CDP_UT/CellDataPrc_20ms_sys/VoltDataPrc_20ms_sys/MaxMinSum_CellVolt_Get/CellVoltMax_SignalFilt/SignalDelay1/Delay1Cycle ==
  u : Inport
  Constant2 : Constant  Value=ASWTYPE_FALSE
  Switch : Switch  Criteria=u2 ~= 0  Threshold=1  RndMeth=Zero
  Unit Delay1 : UnitDelay  SampleTime=-1  StateName=StateName
  Unit Delay21 : UnitDelay  InitialCondition=1  SampleTime=-1  StateName=StateName
  y : Outport
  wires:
  Switch/1 -> y/1
  u/1 -> Switch/1, Unit Delay1/1
  Unit Delay1/1 -> Switch/3
  Unit Delay21/1 -> Switch/2
  Constant2/1 -> Unit Delay21/1

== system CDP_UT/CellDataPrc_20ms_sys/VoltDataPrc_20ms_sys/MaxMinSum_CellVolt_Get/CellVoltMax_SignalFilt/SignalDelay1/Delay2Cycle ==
  u : Inport
  Constant2 : Constant  Value=ASWTYPE_FALSE
  Switch : Switch  Criteria=u2 ~= 0  Threshold=1  RndMeth=Zero
  Unit Delay1 : UnitDelay  SampleTime=-1  StateName=StateName
  Unit Delay2 : UnitDelay  InitialCondition=1  SampleTime=-1  StateName=StateName
  Unit Delay21 : UnitDelay  InitialCondition=1  SampleTime=-1  StateName=StateName
  Unit Delay3 : UnitDelay  SampleTime=-1  StateName=StateName
  y : Outport
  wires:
  Unit Delay3/1 -> Switch/3
  Unit Delay2/1 -> Switch/2
  Constant2/1 -> Unit Delay21/1
  Unit Delay21/1 -> Unit Delay2/1
  Unit Delay1/1 -> Unit Delay3/1
  u/1 -> Unit Delay1/1, Switch/1
  Switch/1 -> y/1

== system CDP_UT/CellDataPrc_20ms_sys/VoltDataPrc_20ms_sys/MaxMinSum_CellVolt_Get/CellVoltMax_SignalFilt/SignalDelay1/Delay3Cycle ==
  u : Inport
  Constant2 : Constant  Value=ASWTYPE_FALSE
  Switch : Switch  Criteria=u2 ~= 0  Threshold=1  RndMeth=Zero
  Unit Delay1 : UnitDelay  SampleTime=-1  StateName=StateName
  Unit Delay2 : UnitDelay  InitialCondition=1  SampleTime=-1  StateName=StateName
  Unit Delay21 : UnitDelay  InitialCondition=1  SampleTime=-1  StateName=StateName
  Unit Delay3 : UnitDelay  SampleTime=-1  StateName=StateName
  Unit Delay4 : UnitDelay  InitialCondition=1  SampleTime=-1  StateName=StateName
  Unit Delay5 : UnitDelay  SampleTime=-1  StateName=StateName
  y : Outport
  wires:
  Unit Delay5/1 -> Switch/3
  Unit Delay4/1 -> Switch/2
  Unit Delay3/1 -> Unit Delay5/1
  Unit Delay2/1 -> Unit Delay4/1
  Constant2/1 -> Unit Delay21/1
  Unit Delay21/1 -> Unit Delay2/1
  Unit Delay1/1 -> Unit Delay3/1
  u/1 -> Unit Delay1/1, Switch/1
  Switch/1 -> y/1

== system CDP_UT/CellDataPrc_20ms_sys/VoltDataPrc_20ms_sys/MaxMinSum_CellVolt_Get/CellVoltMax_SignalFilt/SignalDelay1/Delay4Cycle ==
  u : Inport
  Constant2 : Constant  Value=ASWTYPE_FALSE
  Switch : Switch  Criteria=u2 ~= 0  Threshold=1  RndMeth=Zero
  Unit Delay{1,3,5,7} (4 alike) : UnitDelay  SampleTime=-1  StateName=StateName
  Unit Delay{2,4,6,21} (4 alike) : UnitDelay  InitialCondition=1  SampleTime=-1  StateName=StateName
  y : Outport
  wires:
  Unit Delay7/1 -> Switch/3
  Unit Delay6/1 -> Switch/2
  Unit Delay5/1 -> Unit Delay7/1
  Unit Delay4/1 -> Unit Delay6/1
  Unit Delay3/1 -> Unit Delay5/1
  Unit Delay2/1 -> Unit Delay4/1
  Constant2/1 -> Unit Delay21/1
  Unit Delay21/1 -> Unit Delay2/1
  Unit Delay1/1 -> Unit Delay3/1
  u/1 -> Unit Delay1/1, Switch/1
  Switch/1 -> y/1

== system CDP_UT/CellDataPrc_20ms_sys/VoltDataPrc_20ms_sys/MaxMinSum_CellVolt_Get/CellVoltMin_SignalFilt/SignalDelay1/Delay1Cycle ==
  u : Inport
  Constant2 : Constant  Value=ASWTYPE_FALSE
  Switch : Switch  Criteria=u2 ~= 0  Threshold=1  RndMeth=Zero
  Unit Delay1 : UnitDelay  SampleTime=-1  StateName=StateName
  Unit Delay21 : UnitDelay  InitialCondition=1  SampleTime=-1  StateName=StateName
  y : Outport
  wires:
  Constant2/1 -> Unit Delay21/1
  Unit Delay21/1 -> Switch/2
  Unit Delay1/1 -> Switch/3
  u/1 -> Unit Delay1/1, Switch/1
  Switch/1 -> y/1

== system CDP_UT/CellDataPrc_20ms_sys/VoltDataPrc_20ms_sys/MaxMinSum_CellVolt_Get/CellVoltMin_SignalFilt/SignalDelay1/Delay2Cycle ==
  u : Inport
  Constant2 : Constant  Value=ASWTYPE_FALSE
  Switch : Switch  Criteria=u2 ~= 0  Threshold=1  RndMeth=Zero
  Unit Delay1 : UnitDelay  SampleTime=-1  StateName=StateName
  Unit Delay2 : UnitDelay  InitialCondition=1  SampleTime=-1  StateName=StateName
  Unit Delay21 : UnitDelay  InitialCondition=1  SampleTime=-1  StateName=StateName
  Unit Delay3 : UnitDelay  SampleTime=-1  StateName=StateName
  y : Outport
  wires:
  Switch/1 -> y/1
  u/1 -> Switch/1, Unit Delay1/1
  Unit Delay1/1 -> Unit Delay3/1
  Unit Delay21/1 -> Unit Delay2/1
  Constant2/1 -> Unit Delay21/1
  Unit Delay2/1 -> Switch/2
  Unit Delay3/1 -> Switch/3

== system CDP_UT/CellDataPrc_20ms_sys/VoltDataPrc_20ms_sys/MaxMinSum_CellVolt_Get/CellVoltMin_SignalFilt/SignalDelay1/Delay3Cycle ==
  u : Inport
  Constant2 : Constant  Value=ASWTYPE_FALSE
  Switch : Switch  Criteria=u2 ~= 0  Threshold=1  RndMeth=Zero
  Unit Delay1 : UnitDelay  SampleTime=-1  StateName=StateName
  Unit Delay2 : UnitDelay  InitialCondition=1  SampleTime=-1  StateName=StateName
  Unit Delay21 : UnitDelay  InitialCondition=1  SampleTime=-1  StateName=StateName
  Unit Delay3 : UnitDelay  SampleTime=-1  StateName=StateName
  Unit Delay4 : UnitDelay  InitialCondition=1  SampleTime=-1  StateName=StateName
  Unit Delay5 : UnitDelay  SampleTime=-1  StateName=StateName
  y : Outport
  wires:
  Switch/1 -> y/1
  u/1 -> Switch/1, Unit Delay1/1
  Unit Delay1/1 -> Unit Delay3/1
  Unit Delay21/1 -> Unit Delay2/1
  Constant2/1 -> Unit Delay21/1
  Unit Delay2/1 -> Unit Delay4/1
  Unit Delay3/1 -> Unit Delay5/1
  Unit Delay4/1 -> Switch/2
  Unit Delay5/1 -> Switch/3

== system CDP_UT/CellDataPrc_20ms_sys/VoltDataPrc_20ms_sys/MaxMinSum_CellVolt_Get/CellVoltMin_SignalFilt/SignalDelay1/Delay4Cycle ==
  u : Inport
  Constant2 : Constant  Value=ASWTYPE_FALSE
  Switch : Switch  Criteria=u2 ~= 0  Threshold=1  RndMeth=Zero
  Unit Delay{1,3,5,7} (4 alike) : UnitDelay  SampleTime=-1  StateName=StateName
  Unit Delay{2,4,6,21} (4 alike) : UnitDelay  InitialCondition=1  SampleTime=-1  StateName=StateName
  y : Outport
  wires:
  Switch/1 -> y/1
  u/1 -> Switch/1, Unit Delay1/1
  Unit Delay1/1 -> Unit Delay3/1
  Unit Delay21/1 -> Unit Delay2/1
  Constant2/1 -> Unit Delay21/1
  Unit Delay2/1 -> Unit Delay4/1
  Unit Delay3/1 -> Unit Delay5/1
  Unit Delay4/1 -> Unit Delay6/1
  Unit Delay5/1 -> Unit Delay7/1
  Unit Delay6/1 -> Switch/2
  Unit Delay7/1 -> Switch/3

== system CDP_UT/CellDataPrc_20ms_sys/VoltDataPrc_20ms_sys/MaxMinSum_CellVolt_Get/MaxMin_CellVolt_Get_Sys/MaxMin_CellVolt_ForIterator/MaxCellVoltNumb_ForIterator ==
  LcCDP_IniOutputCellVolt_mV : Inport
  LcCDP_IniOutputCellVoltNumb_numb : Inport  Port=2
  LbCDP_IniOutputCellVoltVld_flg : Inport  Port=3
  Logical Operator : Logic  AllPortsSameDT=off  OutDataTypeStr=boolean
  Relational Operator3 : RelationalOperator  Operator=<=  OutDataTypeStr=boolean
  Switch : Switch  Criteria=u2 ~= 0
  Switch1 : Switch  Criteria=u2 ~= 0
  Unit Delay : UnitDelay  SampleTime=-1  StateName=StateName
  Unit Delay External IC1 : AIWAYS_Powertrain_BMS_lib/Delay Blocks/Unit Delay External IC
  Unit Delay1 : UnitDelay  SampleTime=-1  StateName=StateName
  LcCDP_MaxCellVolt_mV : Outport
  LcCDP_MaxCellVoltNumb_numb : Outport  Port=2
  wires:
  Switch/1 -> Unit Delay External IC1/1, LcCDP_MaxCellVolt_mV/1, Unit Delay/1  "LcCDP_MaxCellVolt_mV"
  LcCDP_IniOutputCellVoltNumb_numb/1 -> Switch1/1
  Unit Delay1/1 -> Switch1/3
  Unit Delay External IC1/1 -> Relational Operator3/1
  Unit Delay/1 -> Switch/3
  Switch1/1 -> Unit Delay1/1, LcCDP_MaxCellVoltNumb_numb/1  "LcCDP_MaxCellVoltNumb_numb"
  LcCDP_IniOutputCellVolt_mV/1 -> Switch/1, Relational Operator3/2, Unit Delay External IC1/2
  Relational Operator3/1 -> [LbCDP_CellVoltMaxCondition_flg]  "LbCDP_CellVoltMaxCondition_flg"
  [LbCDP_CellVoltMaxCondition_flg] -> Logical Operator/1
  LbCDP_IniOutputCellVoltVld_flg/1 -> Logical Operator/2
  Logical Operator/1 -> Switch1/2, Switch/2

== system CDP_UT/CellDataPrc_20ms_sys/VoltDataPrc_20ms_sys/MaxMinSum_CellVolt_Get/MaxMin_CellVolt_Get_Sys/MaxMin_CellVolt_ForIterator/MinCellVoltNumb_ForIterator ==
  LcCDP_IniOutputCellVolt_mV : Inport
  LcCDP_IniOutputCellVoltNumb_numb : Inport  Port=2
  LbCDP_IniOutputCellVoltVld_flg : Inport  Port=3
  Constant3 : Constant  Value=CcCDP_MinVoltIniVal_mV
  Logical Operator : Logic  AllPortsSameDT=off  OutDataTypeStr=boolean
  Relational Operator3 : RelationalOperator  OutDataTypeStr=boolean
  Switch : Switch  Criteria=u2 ~= 0
  Switch1 : Switch  Criteria=u2 ~= 0
  Unit Delay External IC1 : AIWAYS_Powertrain_BMS_lib/Delay Blocks/Unit Delay External IC
  Unit Delay External IC2 : AIWAYS_Powertrain_BMS_lib/Delay Blocks/Unit Delay External IC
  Unit Delay1 : UnitDelay  SampleTime=-1  StateName=StateName
  LcCDP_MinCellVolt_mV : Outport
  LcCDP_MinCellVoltNumb_numb : Outport  Port=2
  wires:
  LcCDP_IniOutputCellVolt_mV/1 -> Switch/1, Relational Operator3/2, Unit Delay External IC1/2
  Unit Delay External IC2/1 -> Switch/3
  Unit Delay1/1 -> Switch1/3
  Relational Operator3/1 -> [LbCDP_CellVoltMinCondition_flg]  "LbCDP_CellVoltMinCondition_flg"
  LcCDP_IniOutputCellVoltNumb_numb/1 -> Switch1/1
  Unit Delay External IC1/1 -> Relational Operator3/1
  Switch1/1 -> LcCDP_MinCellVoltNumb_numb/1, Unit Delay1/1  "LcCDP_MinCellVoltNumb_numb"
  Switch/1 -> Unit Delay External IC2/1, Unit Delay External IC1/1, LcCDP_MinCellVolt_mV/1  "LcCDP_MinCellVolt_mV"
  [LbCDP_CellVoltMinCondition_flg] -> Logical Operator/1
  LbCDP_IniOutputCellVoltVld_flg/1 -> Logical Operator/2
  Logical Operator/1 -> Switch1/2, Switch/2
  Constant3/1 -> Unit Delay External IC2/2

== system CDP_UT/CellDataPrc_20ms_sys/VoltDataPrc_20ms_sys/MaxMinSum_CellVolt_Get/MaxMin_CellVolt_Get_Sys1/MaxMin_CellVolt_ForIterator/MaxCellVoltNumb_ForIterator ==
  LcCDP_IniOutputCellVolt_mV : Inport
  LcCDP_IniOutputCellVoltNumb_numb : Inport  Port=2
  LbCDP_IniOutputCellVoltVld_flg : Inport  Port=3
  Logical Operator : Logic  AllPortsSameDT=off  OutDataTypeStr=boolean
  Relational Operator3 : RelationalOperator  Operator=<=  OutDataTypeStr=boolean
  Switch : Switch  Criteria=u2 ~= 0
  Switch1 : Switch  Criteria=u2 ~= 0
  Unit Delay : UnitDelay  SampleTime=-1  StateName=StateName
  Unit Delay External IC1 : AIWAYS_Powertrain_BMS_lib/Delay Blocks/Unit Delay External IC
  Unit Delay1 : UnitDelay  SampleTime=-1  StateName=StateName
  LcCDP_MaxCellVolt_mV : Outport
  LcCDP_MaxCellVoltNumb_numb : Outport  Port=2
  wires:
  Logical Operator/1 -> Switch/2, Switch1/2
  LbCDP_IniOutputCellVoltVld_flg/1 -> Logical Operator/2
  [LbCDP_CellVoltMaxCondition_flg] -> Logical Operator/1
  Relational Operator3/1 -> [LbCDP_CellVoltMaxCondition_flg]  "LbCDP_CellVoltMaxCondition_flg"
  LcCDP_IniOutputCellVolt_mV/1 -> Unit Delay External IC1/2, Relational Operator3/2, Switch/1
  Switch1/1 -> LcCDP_MaxCellVoltNumb_numb/1, Unit Delay1/1  "LcCDP_MaxCellVoltNumb_numb"
  Unit Delay/1 -> Switch/3
  Unit Delay External IC1/1 -> Relational Operator3/1
  Unit Delay1/1 -> Switch1/3
  LcCDP_IniOutputCellVoltNumb_numb/1 -> Switch1/1
  Switch/1 -> Unit Delay/1, LcCDP_MaxCellVolt_mV/1, Unit Delay External IC1/1  "LcCDP_MaxCellVolt_mV"

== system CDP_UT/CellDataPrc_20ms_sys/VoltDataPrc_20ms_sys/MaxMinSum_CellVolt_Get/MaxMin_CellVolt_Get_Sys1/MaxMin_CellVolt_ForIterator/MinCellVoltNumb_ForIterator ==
  LcCDP_IniOutputCellVolt_mV : Inport
  LcCDP_IniOutputCellVoltNumb_numb : Inport  Port=2
  LbCDP_IniOutputCellVoltVld_flg : Inport  Port=3
  Constant3 : Constant  Value=CcCDP_MinVoltIniVal_mV
  Logical Operator : Logic  AllPortsSameDT=off  OutDataTypeStr=boolean
  Relational Operator3 : RelationalOperator  OutDataTypeStr=boolean
  Switch : Switch  Criteria=u2 ~= 0
  Switch1 : Switch  Criteria=u2 ~= 0
  Unit Delay External IC1 : AIWAYS_Powertrain_BMS_lib/Delay Blocks/Unit Delay External IC
  Unit Delay External IC2 : AIWAYS_Powertrain_BMS_lib/Delay Blocks/Unit Delay External IC
  Unit Delay1 : UnitDelay  SampleTime=-1  StateName=StateName
  LcCDP_MinCellVolt_mV : Outport
  LcCDP_MinCellVoltNumb_numb : Outport  Port=2
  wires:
  Constant3/1 -> Unit Delay External IC2/2
  Logical Operator/1 -> Switch/2, Switch1/2
  LbCDP_IniOutputCellVoltVld_flg/1 -> Logical Operator/2
  [LbCDP_CellVoltMinCondition_flg] -> Logical Operator/1
  Switch/1 -> LcCDP_MinCellVolt_mV/1, Unit Delay External IC1/1, Unit Delay External IC2/1  "LcCDP_MinCellVolt_mV"
  Switch1/1 -> Unit Delay1/1, LcCDP_MinCellVoltNumb_numb/1  "LcCDP_MinCellVoltNumb_numb"
  Unit Delay External IC1/1 -> Relational Operator3/1
  LcCDP_IniOutputCellVoltNumb_numb/1 -> Switch1/1
  Relational Operator3/1 -> [LbCDP_CellVoltMinCondition_flg]  "LbCDP_CellVoltMinCondition_flg"
  Unit Delay1/1 -> Switch1/3
  Unit Delay External IC2/1 -> Switch/3
  LcCDP_IniOutputCellVolt_mV/1 -> Unit Delay External IC1/2, Relational Operator3/2, Switch/1

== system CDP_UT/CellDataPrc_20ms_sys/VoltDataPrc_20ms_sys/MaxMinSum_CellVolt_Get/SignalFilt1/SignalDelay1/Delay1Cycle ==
  u : Inport
  Constant2 : Constant  Value=ASWTYPE_FALSE
  Switch : Switch  Criteria=u2 ~= 0  Threshold=1  RndMeth=Zero
  Unit Delay1 : UnitDelay  SampleTime=-1  StateName=StateName
  Unit Delay21 : UnitDelay  InitialCondition=1  SampleTime=-1  StateName=StateName
  y : Outport
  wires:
  Constant2/1 -> Unit Delay21/1
  Unit Delay21/1 -> Switch/2
  Unit Delay1/1 -> Switch/3
  u/1 -> Unit Delay1/1, Switch/1
  Switch/1 -> y/1

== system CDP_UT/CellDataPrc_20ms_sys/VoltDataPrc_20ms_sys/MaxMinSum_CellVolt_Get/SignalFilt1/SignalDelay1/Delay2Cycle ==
  u : Inport
  Constant2 : Constant  Value=ASWTYPE_FALSE
  Switch : Switch  Criteria=u2 ~= 0  Threshold=1  RndMeth=Zero
  Unit Delay1 : UnitDelay  SampleTime=-1  StateName=StateName
  Unit Delay2 : UnitDelay  InitialCondition=1  SampleTime=-1  StateName=StateName
  Unit Delay21 : UnitDelay  InitialCondition=1  SampleTime=-1  StateName=StateName
  Unit Delay3 : UnitDelay  SampleTime=-1  StateName=StateName
  y : Outport
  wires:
  Switch/1 -> y/1
  u/1 -> Switch/1, Unit Delay1/1
  Unit Delay1/1 -> Unit Delay3/1
  Unit Delay21/1 -> Unit Delay2/1
  Constant2/1 -> Unit Delay21/1
  Unit Delay2/1 -> Switch/2
  Unit Delay3/1 -> Switch/3

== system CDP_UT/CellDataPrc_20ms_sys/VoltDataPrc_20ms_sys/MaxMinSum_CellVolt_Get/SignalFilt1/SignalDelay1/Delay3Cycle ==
  u : Inport
  Constant2 : Constant  Value=ASWTYPE_FALSE
  Switch : Switch  Criteria=u2 ~= 0  Threshold=1  RndMeth=Zero
  Unit Delay1 : UnitDelay  SampleTime=-1  StateName=StateName
  Unit Delay2 : UnitDelay  InitialCondition=1  SampleTime=-1  StateName=StateName
  Unit Delay21 : UnitDelay  InitialCondition=1  SampleTime=-1  StateName=StateName
  Unit Delay3 : UnitDelay  SampleTime=-1  StateName=StateName
  Unit Delay4 : UnitDelay  InitialCondition=1  SampleTime=-1  StateName=StateName
  Unit Delay5 : UnitDelay  SampleTime=-1  StateName=StateName
  y : Outport
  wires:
  Switch/1 -> y/1
  u/1 -> Switch/1, Unit Delay1/1
  Unit Delay1/1 -> Unit Delay3/1
  Unit Delay21/1 -> Unit Delay2/1
  Constant2/1 -> Unit Delay21/1
  Unit Delay2/1 -> Unit Delay4/1
  Unit Delay3/1 -> Unit Delay5/1
  Unit Delay4/1 -> Switch/2
  Unit Delay5/1 -> Switch/3

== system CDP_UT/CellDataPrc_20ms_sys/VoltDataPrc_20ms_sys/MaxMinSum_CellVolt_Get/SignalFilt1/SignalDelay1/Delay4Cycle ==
  u : Inport
  Constant2 : Constant  Value=ASWTYPE_FALSE
  Switch : Switch  Criteria=u2 ~= 0  Threshold=1  RndMeth=Zero
  Unit Delay{1,3,5,7} (4 alike) : UnitDelay  SampleTime=-1  StateName=StateName
  Unit Delay{2,4,6,21} (4 alike) : UnitDelay  InitialCondition=1  SampleTime=-1  StateName=StateName
  y : Outport
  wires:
  Switch/1 -> y/1
  u/1 -> Switch/1, Unit Delay1/1
  Unit Delay1/1 -> Unit Delay3/1
  Unit Delay21/1 -> Unit Delay2/1
  Constant2/1 -> Unit Delay21/1
  Unit Delay2/1 -> Unit Delay4/1
  Unit Delay3/1 -> Unit Delay5/1
  Unit Delay4/1 -> Unit Delay6/1
  Unit Delay5/1 -> Unit Delay7/1
  Unit Delay6/1 -> Switch/2
  Unit Delay7/1 -> Switch/3
